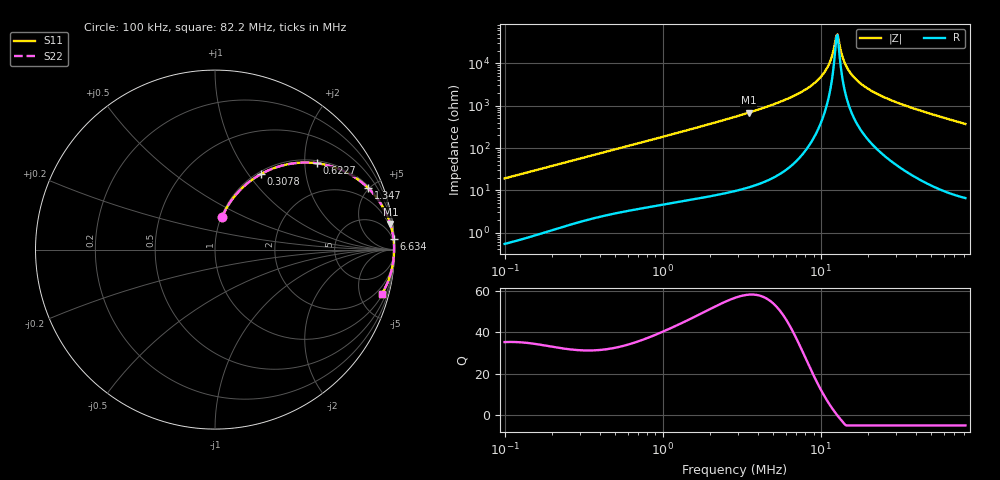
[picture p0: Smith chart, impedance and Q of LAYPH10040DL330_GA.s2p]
! LAYPH10040DL330_GA  S-PARAMETER MODEL  ( General Type )
! Model Generated by TAIYO YUDEN Corporation (http://www.ty-top.com)
! Version 1.0
! TAIYO YUDEN Control No. 180920NI43SB-FBB
! Copyright(c) 2018 TAIYO YUDEN CO.,LTD. All Rights Reserved.
! Product Description (link to TY-COMPAS)
! https://ds.yuden.co.jp/TYCOMPAS/or/detail?pn=LAYPH10040DL330MGA&u=M
! Products Name : Inductors
! Characteristics :
!  Inductance : 33 uH , SRF(min) : -Hz , DC Resistance(max) : 0.115 Ohm
!  Rated Current : Saturation :2 A , Temp Rise : 1.1 A (25 degC)
!  Case Size : 10.1 x 10.0 / 0.398 x 0.394 [mm/inch] , Thickness : 4 / 0.157 [mm/inch]
!  (Conditions: Temperature = 25 degC , DC Bias Current/Voltage = 0A / 0V)
! External Node Assignments :
!  1  o---GGG---o  2
! GND o---------o GND
! Frequency Range : 0.1MHz  -  82.198079MHz  [ 402 STEP ]
# MHz S RI R 50
! Freq[MHz].  S11 Real  S11 Imag  S21 Real  S21 Imag  S12 Real  S12 Imag  S22 Real  S22 Imag
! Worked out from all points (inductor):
!   401 points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, 100 kHz to 82.2 MHz, reference 50 ohm
!   read as one part in series: L = 30.3 uH near 103.4 kHz
!   highest Q = 58.3 at 3.507 MHz (marker M1), where L = 31.1 uH
!   self-resonance near 12.55 MHz
!   S11 on the Smith chart (normalised r, x): 100 kHz: 1.01, +0.38; 307.8 kHz: 1.04, +1.15; 622.7 kHz: 1.07, +2.30; 1.347 MHz: 1.11, +4.96; 6.634 MHz: 2, +33; 82.2 MHz: 1.13, -7.40
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0.1  0.0401 0.1826  0.9599 -0.1826  0.9599 -0.1826  0.0401 0.1826
0.182952  0.1145 0.3039  0.8855 -0.3039  0.8855 -0.3039  0.1145 0.3039
0.307779  0.2567 0.4211  0.7433 -0.4211  0.7433 -0.4211  0.2567 0.4211
0.62273  0.5675 0.4811  0.4325 -0.4811  0.4325 -0.4811  0.5675 0.4811
0.947281  0.7466 0.4225  0.2534 -0.4225  0.2534 -0.4225  0.7466 0.4225
1.347438  0.8546 0.3416  0.1454 -0.3416  0.1454 -0.3416  0.8546 0.3416
2.867021  0.9646 0.1762  0.0354 -0.1762  0.0354 -0.1762  0.9646 0.1762
3.506523  0.9768 0.1422  0.0232 -0.1422  0.0232 -0.1422  0.9768 0.1422
6.6342  0.9949 0.0602  0.00513 -0.0602  0.00513 -0.0602  0.9949 0.0602
8.824095  0.9974 0.0321  0.0026 -0.0321  0.0026 -0.0321  0.9974 0.0321
9.923851  0.9979 0.0214  0.00214 -0.0214  0.00214 -0.0214  0.9979 0.0214
10.97497  0.998 0.0126  0.00196 -0.0126  0.00196 -0.0126  0.998 0.0126
11.73686  0.9981 0.00673  0.00194 -0.00673  0.00194 -0.00673  0.9981 0.00673
12.34279  0.998 0.0024  0.00197 -0.0024  0.00197 -0.0024  0.998 0.0024
12.76402  0.998 -0.000483  0.00201 0.000483  0.00201 0.000483  0.998 -0.000483
12.98  0.998 -0.00192  0.00204 0.00192  0.00204 0.00192  0.998 -0.00192
13.65011  0.9979 -0.00623  0.00215 0.00623  0.00215 0.00623  0.9979 -0.00623
14.35482  0.9977 -0.0105  0.00228 0.0105  0.00228 0.0105  0.9977 -0.0105
16.14387  0.9973 -0.0207  0.00274 0.0207  0.00274 0.0207  0.9973 -0.0207
19.74484  0.996 -0.0387  0.00399 0.0387  0.00399 0.0387  0.996 -0.0387
27.15873  0.9923 -0.0706  0.0077 0.0706  0.0077 0.0706  0.9923 -0.0706
82.19808  0.9281 -0.2496  0.0719 0.2496  0.0719 0.2496  0.9281 -0.2496
